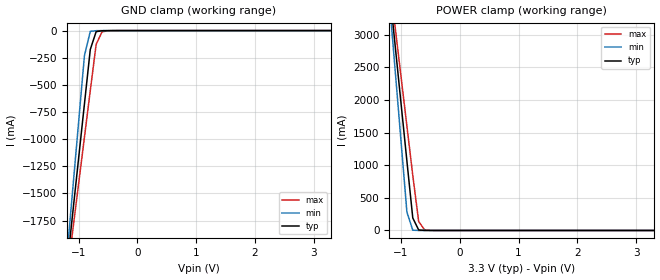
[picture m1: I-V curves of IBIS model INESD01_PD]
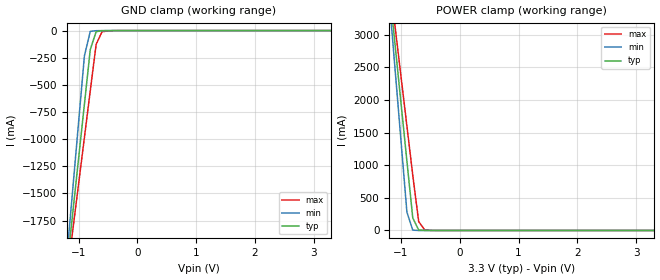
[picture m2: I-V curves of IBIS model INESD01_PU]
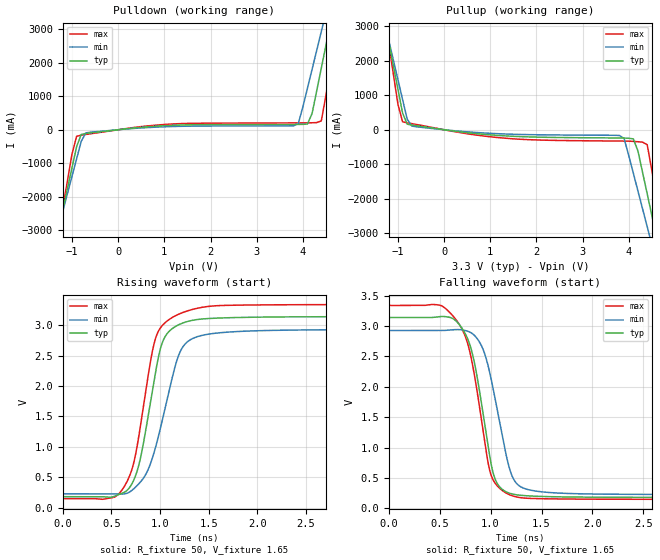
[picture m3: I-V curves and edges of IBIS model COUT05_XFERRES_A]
|   This file is an IBIS representation of the   |
|   Integrated Devices Technology, Inc.   |
|   ICS83026I   |
|   LOW SKEW, 1-TO-2 DIFFERENTIAL-TO-LVCMOS/LVTTL FANOUT BUFFER   |
[IBIS Ver]   4.1
[File name]   83026i__3v3.ibs
[File Rev]   0.0
[Date]   29 Apr 2009 | Last modified
|   Aug 22 2003 | Generated
[Source]   Originated at Integrated Devices Technology, Inc.
[Disclaimer]
IDT hereby grants the user of this IBIS model a non-exclusive,
nontransferable license to use this IBIS model under the following terms.
Before using this IBIS model, the user should read this license.
If the user does not accept these terms,  the IBIS model should be
returned to IDT within 30 days.
   The user is granted this license only to use the IBIS model and
is not granted rights to sell, load, rent, lease or license the IBIS
model in whole or in part, or in modified form to anyone other than
user. User may modify the IBIS model to suit its specific
applications but rights to derivative works and such modifications
shall belong to IDT.
   This IBIS model is provided on an "AS IS" basis and IDT makes
absolutely no warranty with respect to the information contained
herein. IDT DISCLAIMS AND CUSTOMER WAIVES ALL WARRANTIES, EXPRESS
OR IMPLIED, INCLUDING WARRANTIES OF MERCHANTABILITY OR FITNESS FOR
A PARTICULAR PURPOSE. The entire risk as to quality and performance
is with the Customer. ACCORDINGLY, IN NO EVENT SHALL THE COMPANY BE
LIABLE FOR ANY DAMAGES, WHETHER IN CONTRACT OR TORT,INCLUDING ANY
LOST PROFITS OR OTHER INCIDENTAL, CONSEQUENTIAL, EXEMPLARY, OR
PUNITIVE DAMAGES ARISING OUT OF THE USE OR APPLICATION OF THE IBIS
model provided in this package. Further, IDT reserves the right to
make changes without notice to any product herein to improve
reliability, function, or design. IDT does not convey any license
under patent rights or any other intellectual property rights,
including those of third parties.
   IDT is not obligated to provide maintenance or support
for the licensed IBIS model.
[Copyright]   Copyright 2003 by Integrated Devices Technology, Inc.
[Component]   ICS83026MI
[Manufacturer] Integrated Devices Technology, Inc.
[Package]
|SOIC 8 Lead
|   typ   min   max
R_pkg   57.05m   55.5m   58.6m
L_pkg   1.769nH   1.570nH   1.968nH
C_pkg   0.269pF   0.252pF   0.286pF
[Pin]   signal_name   model_name   R_pin   L_pin   C_pin
1   NC   NC   58.6m   1.968n   0.286p
2   CLK   INESD01_PD   55.5m   1.570n   0.252p
3   nCLK   INESD01_PU   55.5m   1.570n   0.252p
4   NC   NC   56.6m   1.968n   0.286p
5   GND   GND   58.6m   1.968n   0.286p
6   Q1   COUT05_XFERRES_A   55.5m   1.570n   0.252p
7   Q0   COUT05_XFERRES_A   55.5m   1.570n   0.252p
8   VDD   POWER   56.6m   1.968n   0.286p
[Diff Pin]   inv_pin  vdiff tdelay_typ tdelay_min  tdelay_max
2   3   NA   0   0   0
| Models and submodels in the file (3): INESD01_PD (Input), INESD01_PU (Input), COUT05_XFERRES_A (Output)
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[Model]   INESD01_PD
Model_type   Input
Polarity   Non-Inverting
Vinl = 0.80V
Vinh = 2.0V
|   typ   min   max
C_comp   2pF   1.5pF   2.5pF
|   typ   min   max
[Voltage range]  3.3V   3.15V   3.45V
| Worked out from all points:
|   GND clamp passes 1 mA (typ) near -0.55 V on its own axis
|   POWER clamp passes 1 mA (typ) near -0.60 V on its own axis
[GND_clamp]
|Voltage I(typ)   I(min)   I(max)
-3.3V     -12.83A    -15.14A    -11.37A
-1.2V     -2.195A    -2.092A    -2.281A
-1.1V     -1.689A    -1.472A    -1.849A
-900mV    -678.5mA   -232.6mA   -984.8mA
-800mV    -173.9mA   -7.175mA   -553.2mA
-700mV    -9.696mA   -1.052mA   -126mA
-600mV    -1.629mA   -178uA     -11.07mA
-300mV    -10.53uA   -5.678uA   -86.08uA
3.3V      71.13uA    62.11uA    77.58uA
[POWER_clamp]
|Voltage   I(typ)   I(min)   I(max)
-3.3V     22.38A     26.45A     19.82A
-1.2V     3.723A     3.545A     3.874A
-1.1V     2.836A     2.457A     3.116A
-1V       1.949A     1.369A     2.358A
-900mV    1.063A     281.1mA    1.601A
-800mV    191.6mA    5.074mA    844mA
-700mV    8.104mA    204.3uA    138.4mA
-600mV    678.1uA    79.74uA    10.7mA
-400mV    87.44uA    69.65uA    413.2uA
3.3V      -3.041nA   -425fA     -919.9nA
[Model]   INESD01_PU
Model_type   Input
Polarity   Non-Inverting
Vinl = 0.8V
Vinh = 2.0V
|   typ   min   max
C_comp   2pF   1.5pF   2.5pF
|   typ   min   max
[Voltage range]  3.3V   3.15V   3.45V
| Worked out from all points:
|   GND clamp passes 1 mA (typ) near -0.55 V on its own axis
|   POWER clamp passes 1 mA (typ) near -0.61 V on its own axis
[GND_clamp]
|Voltage   I(typ)   I(min)   I(max)
-3.3V     -12.83A    -15.14A    -11.37A
-1.2V     -2.195A    -2.092A    -2.281A
-1.1V     -1.689A    -1.472A    -1.849A
-900mV    -678.5mA   -232.7mA   -984.8mA
-800mV    -174mA     -7.237mA   -553.3mA
-700mV    -9.767mA   -1.114mA   -126.1mA
-600mV    -1.7mA     -240.1uA   -11.15mA
-300mV    -81.66uA   -67.79uA   -163.4uA
3.3V      1.866nA    1.113pA    239.1nA
[POWER_clamp]
|Voltage   I(typ)   I(min)   I(max)
-3.3V     22.38A     26.45A     19.82A
-1.2V     3.723A     3.545A     3.874A
-1.1V     2.836A     2.457A     3.116A
-1V       1.949A     1.369A     2.358A
-900mV    1.063A     281mA      1.601A
-800mV    191.5mA    5.012mA    843.9mA
-700mV    8.032mA    142.2uA    138.3mA
-600mV    607uA      17.63uA    10.62mA
-400mV    16.32uA    7.545uA    335.9uA
3.3V      -71.13uA   -62.11uA   -78.26uA
[Model]   COUT05_XFERRES_A
Model_type   Output
Polarity   Non-Inverting
|   typ   min   max
C_comp   2pF   1.5pF   2.5pF
Vmeas = 1.75V
Rref = 50
Vref = 1.65V
|   typ   min   max
[Voltage range]   3.3V   3.135V   3.465V
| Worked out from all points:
|   slope of the pulldown table from 0 to 0.495 V, typ, clamps not added: 6.88 ohm
|   slope of the pullup table from 0 to 0.495 V, typ, clamps not added: 5.83 ohm
|   rising waveform, R_fixture 50, V_fixture 1.65: 20-80 % time 201ps typ, 255ps min, 203ps max; typ from 0.181 V to 3.14 V
|   falling waveform, R_fixture 50, V_fixture 1.65: 20-80 % time 180ps typ, 198ps min, 195ps max; typ from 3.14 V to 0.181 V
[pulldown]
|Voltage   I (typ)   I (min)   I (max)
-3.3V     -15.53A    -13.39A    -19.08A
-1.3V     -3.015A    -2.955A    -3.131A
-1V       -1.131A    -1.388A    -725.6mA
-800mV    -139.2mA   -344.2mA   -162.8mA
200mV     32.31mA    23.73mA    41.9mA
3.9V      159.3mA    180.5mA    204.1mA
4.2V      482.4mA    1.8A       208mA
4.4V      1.836A     2.927A     263.7mA
4.6V      3.193A     4.056A     1.89A
4.7V      3.873A     4.622A     2.759A
4.8V      4.554A     5.188A     3.63A
6.6V      17.06A     15.56A     19.6A
[pullup]
|Voltage   I (typ)   I (min)   I (max)
-3.3V     16.98A     14.61A     20.9A
-1.3V     3.243A     3.171A     3.379A
-1V       1.177A     1.453A     739.5mA
-800mV    162.5mA    308.2mA    200.5mA
3.8V      -238.9mA   -166.8mA   -327.9mA
3.9V      -241.3mA   -257.1mA   -328.9mA
4.1V      -265.6mA   -1.266A    -337.6mA
4.4V      -1.864A    -2.816A    -435.8mA
4.6V      -3.109A    -3.852A    -1.975A
4.7V      -3.731A    -4.37A     -2.771A
4.8V      -4.354A    -4.888A    -3.566A
6.6V      -15.57A    -14.23A    -17.87A
[Ramp]
|   typ   min   max
dV/dt_r   2.374/0.330n   2.163/0.407n   2.561/0.368n
dV/dt_f   2.381/0.289n   2.171/0.307n   2.565/0.334n
[Rising Waveform]
R_fixture = 50
V_fixture = 1.65
V_fixture_max = 1.73
V_fixture_min = 1.57
C_fixture = 0.0p
| Time   typ   min   max
0s        180.7mV    228.1mV    148.5mV
524.8ps   184.1mV    227.8mV    170.1mV
697ps     355.4mV    267.5mV    563.7mV
799.5ps   819.2mV    423.5mV    1.35V
947.1ps   2.168V     952.1mV    2.747V
1.033ns   2.751V     1.504V     3.011V
1.16ns    2.979V     2.351V     3.156V
1.279ns   3.059V     2.722V     3.233V
1.542ns   3.112V     2.862V     3.315V
3.997ns   3.14V      2.927V     3.339V
[Falling Waveform]
R_fixture = 50
V_fixture = 1.65
V_fixture_max = 1.73
V_fixture_min = 1.57
C_fixture = 0.0p
| Time   typ   min   max
0s        3.141V     2.927V     3.339V
508.4ps   3.157V     2.927V     3.341V
717.5ps   2.969V     2.938V     2.958V
836.4ps   2.438V     2.854V     2.242V
996.3ps   814.4mV    2.2V       594.2mV
1.062ns   419.3mV    1.65V      376.2mV
1.177ns   254.8mV    710.3mV    231.3mV
1.275ns   218.5mV    378.8mV    180.8mV
1.513ns   195.2mV    270mV      158.2mV
3.997ns   180.7mV    228.1mV    148.5mV
